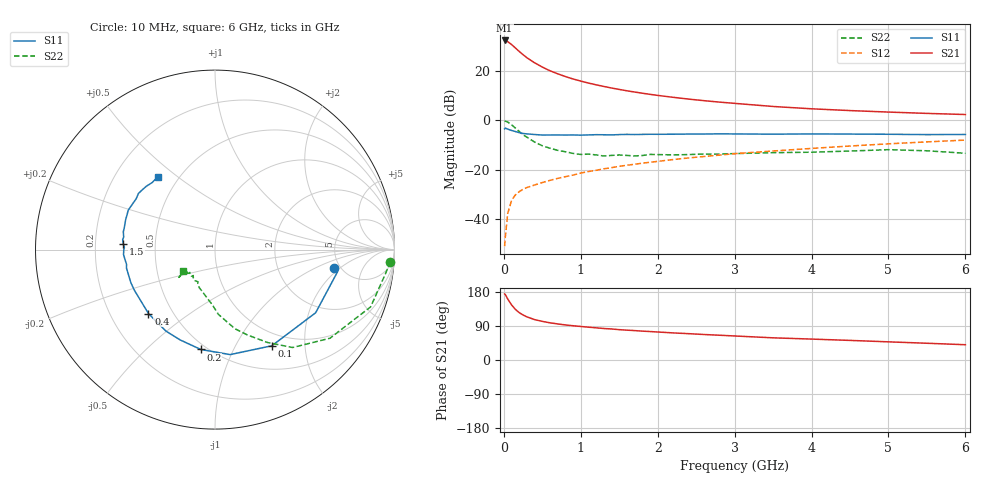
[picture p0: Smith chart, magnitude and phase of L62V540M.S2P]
!  INFINEON TECHNOLOGIES Small Signal Semiconductors
! BFR380L3 , Si-NPN RF-Transistor in TSLP-3-1
!  Vce=2.5 V,  Ic=40 mA
! Common Emitter S-Parameters:  07. March 2005
#  GHz  S  MA  R  50
! f  S11  S21  S12  S22
! GHz  Mag  Ang  Mag  Ang  Mag  Ang  Mag  Ang
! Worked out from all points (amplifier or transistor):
!   36 points, 10 MHz to 6 GHz, reference 50 ohm
!   highest |S21| = 32.4 dB at 10 MHz (marker M1)
!   |S21| within 3 dB of that: start of sweep to 148.7 MHz
!   unconditionally stable (mu >= 1): 1.614 GHz to 4.83 GHz
!   at 250 MHz: K = 0.46, MSG = 27.3 dB, |S12| = -28.0 dB
!   at 1.4 GHz: K = 0.98, MSG = 16.1 dB, |S12| = -19.2 dB
!   at 6 GHz: K = 0.98, MSG = 5.2 dB, |S12| = -8.0 dB
!   S11 on the Smith chart (normalised r, x): 10 MHz: 4.39, -1.67; 100 MHz: 0.81, -1.42; 200 MHz: 0.46, -0.75; 400 MHz: 0.37, -0.36; 1.5 GHz: 0.32, +0.03; 6 GHz: 0.39, +0.43
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0.01  0.67 -9.0  41.55 174.3  0.0028 77.4  0.9797 -3.9
0.02  0.6936 -10.3  41.25 172.4  0.0044 85.6  0.9587 -8.2
0.05  0.662 -32.1  39.34 161.1  0.0128 76.0  0.9239 -20.2
0.1  0.6224 -59.4  34.39 145.5  0.0236 67.1  0.809 -37.6
0.15  0.5911 -81.8  29.3 133.6  0.0307 58.7  0.6961 -51.6
0.2  0.562 -98.1  24.85 125.0  0.0357 56.2  0.5938 -60.6
0.25  0.5394 -111.1  21.39 118.8  0.0399 53.9  0.5072 -69.4
0.3  0.53 -121.1  18.55 113.8  0.0433 53.2  0.4543 -75.9
0.4  0.5142 -136.1  14.63 106.6  0.0487 53.0  0.3612 -87.0
0.5  0.5021 -146.1  12 101.9  0.0546 55.4  0.3044 -93.3
0.6  0.503 -153.3  10.09 98.1  0.0604 56.8  0.2709 -99.8
0.7  0.5037 -158.5  8.755 95.2  0.0664 58.0  0.2456 -106.3
0.9  0.5037 -168.3  6.87 90.4  0.0774 60.4  0.2129 -116.7
1.1  0.5049 -173.9  5.688 86.6  0.0913 62.7  0.2061 -122.4
1.5  0.5125 176.2  4.221 80.1  0.1166 64.8  0.198 -132.1
1.8  0.5172 170.4  3.54 76.2  0.1349 65.2  0.1928 -137.3
2.2  0.5216 164.2  2.923 71.5  0.1598 65.2  0.199 -139.6
2.8  0.5307 155.7  2.338 65.4  0.1967 65.3  0.2066 -145.5
3.5  0.5226 147.2  1.905 58.5  0.2382 63.2  0.2205 -144.1
4.5  0.5251 141.0  1.573 51.7  0.3007 61.5  0.2379 -143.2
5.5  0.5119 133.1  1.379 44.2  0.3647 57.7  0.2406 -142.9
6  0.5161 128.1  1.308 40.3  0.3965 55.4  0.2144 -145.4
